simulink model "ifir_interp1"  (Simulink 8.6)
settings: Solver=FixedStepDiscrete  SolverMode=SingleTasking  StartTime=0.0  StopTime=10.0  RelTol=1e-3
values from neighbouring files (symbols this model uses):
  delay = 2*nord1/2 + (nord2/2)*M1-1    (= 1535)    [basisband_2.m]    (also in ifir_dezim_1.m = fix((length(himage)-1)/2 + 5*(length(h)-1)/2); ifir_high_2.m = length(d)-1; ifir_interp_1.m = fix((length(h)-1)/2 + (length(himage)-1)/(2*L)))
  h = sinc(n-D)    [frac_delay_0.m]    (also in frac_delay_1.m = h.*hanning(length(h))'; frac_delay_2.m = h.*hanning(length(h))'; ifir_1.m = firpm(nord_exp,[0,fp*L,fs*L,0.5]*2,[1,1,0,0],[1,10]); ifir_dezim_1.m = firpm(nord_exp,[0,fp*L,fsp*L,0.5]*2,[1,1,0,0],[1,10]))
  himage = firpm(60, [0,fp,2.7*fp,0.5]*2, [1,1,0,0],[10,1])    [ifir_1.m]    (also in ifir_dezim_1.m; ifir_interp_1.m)
  hsig = fir1(128, 0.02*2)    [ifir_dezim_1.m]    (also in ifir_interp_1.m)
  L = 3    [farrow_3.m]    (also in farrow_4.m = 480; ifir_1.m = 5; ifir_dezim_1.m = 5; ifir_high1.m = 5)
  Ts = 1/fs    (= 5e-05)    [basisband_1.m]    (also in basisband_2.m = 5e-06; dezimier_1.m = 0.0005; dezimier_11.m = 0.0005; dezimier_2.m = 0.0005)
libraries: dspsigops x1

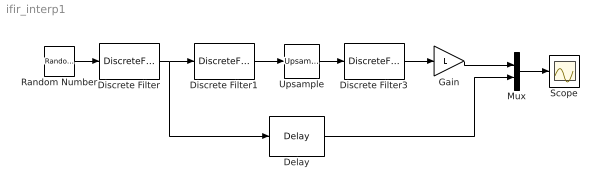
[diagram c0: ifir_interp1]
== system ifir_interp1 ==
  Delay : Delay  DelayLength=delay  InitialCondition=0  InputProcessing=Inherited
  Discrete Filter : DiscreteFilter  Numerator=[hsig]  Denominator=[1 ]  SampleTime=Ts
  Discrete Filter1 : DiscreteFilter  Numerator=[h]  Denominator=[1 ]  SampleTime=Ts
  Discrete Filter3 : DiscreteFilter  Numerator=[himage]  Denominator=[1 ]  SampleTime=Ts/L
  Gain : Gain  Gain=L
  Mux : Mux  Inputs=2
  Random Number : RandomNumber  SampleTime=Ts
  Scope : Scope
  Upsample : dspsigops/Upsample  N=L  phase=0  InputProcessing=Inherited (this choice will be removed - see release notes)  RateOptions=Allow multirate processing  ic=0  mode=Unused parameter value
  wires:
  Random Number/1 -> Discrete Filter/1
  Discrete Filter/1 -> Delay/1, Discrete Filter1/1
  Discrete Filter1/1 -> Upsample/1
  Upsample/1 -> Discrete Filter3/1
  Discrete Filter3/1 -> Gain/1
  Delay/1 -> Mux/2
  Mux/1 -> Scope/1
  Gain/1 -> Mux/1
